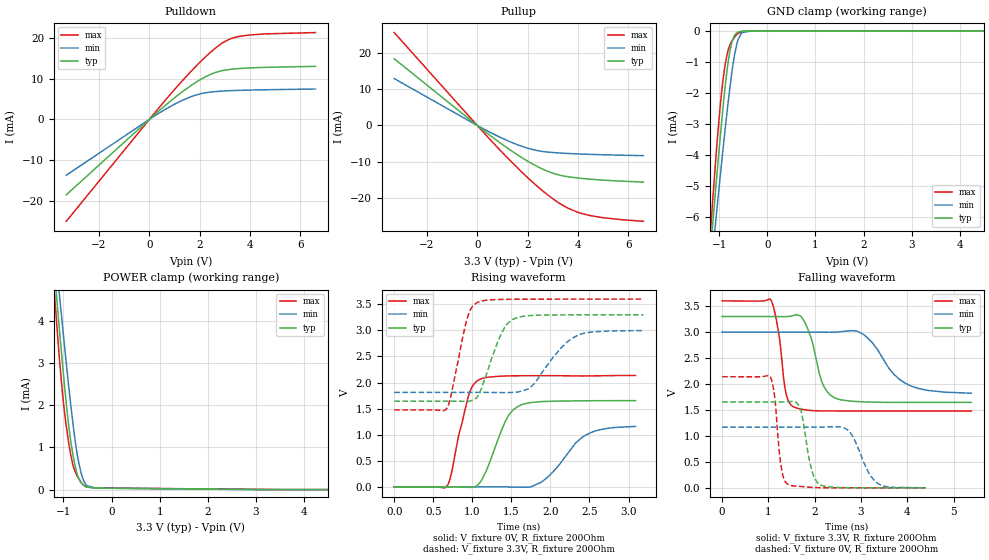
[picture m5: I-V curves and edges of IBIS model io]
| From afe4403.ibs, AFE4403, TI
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|   io Model
[Model]   io
Model_type   I/O
Polarity   Non-Inverting
Enable   Active-Low
Vinl = 0.66
Vinh = 2.64
Vmeas = 1.65
Vref = 0
Cref = 2pF
Rref = 370
|   typ   min   max
|   (nom PVT)   (fast PVT)   (slow PVT)
C_comp   3.788e-13   3.524e-13   3.882e-13
[Model spec]
|subparameter
Vinl   0.66   0.6   0.72
Vinh   2.64   2.4   2.88
| Where nom  PVT is Nominal Process, 3.3V, 27C
|   Fast PVT is Strong Process,  3.6V, -40C
|   Slow PVT is Weak Process,   3V, 105C
[Voltage Range]   3.3   3   3.6
|Junction Temperature
[Temperature Range]   27   105   -40
[Pullup Reference]   3.3   3   3.6
[Pulldown Reference]   0   0   0
[Power Clamp Reference]   3.3   3   3.6
[GND Clamp Reference]   0   0   0
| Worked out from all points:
|   slope of the pulldown table from 0 to 0.495 V, typ, clamps not added: 183 ohm
|   slope of the pullup table from 0 to 0.495 V, typ, clamps not added: 186 ohm
|   GND clamp passes 1 mA (typ) near -0.81 V on its own axis
|   POWER clamp passes 1 mA (typ) near -0.83 V on its own axis
|   falling waveform, V_fixture 3.3V, R_fixture 200Ohm: 20-80 % time 299ps typ, 612ps min, 179ps max; typ from 3.3 V to 1.65 V
|   rising waveform, V_fixture 0V, R_fixture 200Ohm: 20-80 % time 262ps typ, 392ps min, 189ps max; typ from 0 V to 1.65 V
|   rising waveform, V_fixture 3.3V, R_fixture 200Ohm: 20-80 % time 245ps typ, 372ps min, 177ps max; typ from 1.64 V to 3.3 V
|   falling waveform, V_fixture 0V, R_fixture 200Ohm: 20-80 % time 200ps typ, 352ps min, 133ps max; typ from 1.65 V to 0 V
[Pulldown]
|   Voltage   I(typ)   I(min)   I(max)
-3.3V     -18.51mA   -13.7mA    -25.02mA
63mV      352.9uA    259.5uA    478.3uA
821.7mV   4.409mA    3.145mA    6.077mA
1.296V    6.722mA    4.658mA    9.403mA
1.725V    8.612mA    5.747mA    12.26mA
2.237V    10.51mA    6.554mA    15.41mA
2.649V    11.59mA    6.86mA     17.64mA
3.122V    12.22mA    7.045mA    19.54mA
3.633V    12.53mA    7.161mA    20.46mA
4.609V    12.8mA     7.286mA    21.01mA
6.6V      13.04mA    7.482mA    21.34mA
[GND Clamp]
|   Voltage   I(typ)   I(min)   I(max)
-3.3V     -49.34mA   -43.13mA   -58.15mA
-1.216V   -7.733mA   -8.404mA   -7.228mA
-1.158V   -6.649mA   -7.482mA   -5.945mA
-1.143V   -6.369mA   -7.243mA   -5.618mA
-1.066V   -4.952mA   -6.026mA   -3.997mA
-985.2mV  -3.524mA   -4.778mA   -2.503mA
-888mV    -1.953mA   -3.328mA   -1.197mA
-808.8mV  -941.7uA   -2.222mA   -585.8uA
-741mV    -391.7uA   -1.375mA   -342uA
-607.2mV  -38.31uA   -270.4uA   -81.8uA
-330mV    -3.295uA   -3.637uA   -3.333uA
6.6V      0A         0A         0A
[Pullup]
|   Voltage   I(typ)   I(min)   I(max)
-3.3V     18.32mA    12.88mA    25.52mA
0V        0A         0A         0A
877.8mV   -4.633mA   -3.14mA    -6.576mA
1.52V     -7.721mA   -5.078mA   -11.12mA
2.032V    -9.922mA   -6.294mA   -14.52mA
2.442V    -11.46mA   -6.968mA   -17.05mA
2.904V    -12.86mA   -7.37mA    -19.62mA
3.282V    -13.65mA   -7.563mA   -21.44mA
3.627V    -14.1mA    -7.697mA   -22.79mA
4.151V    -14.55mA   -7.856mA   -24.19mA
5.022V    -15.02mA   -8.05mA    -25.35mA
6.6V      -15.54mA   -8.287mA   -26.32mA
[POWER Clamp]
|   Voltage   I(typ)   I(min)   I(max)
-3.3V     35.6mA     31.69mA    41.16mA
-1.183V   5.11mA     5.779mA    4.576mA
-1.098V   3.974mA    4.776mA    3.298mA
-1.079V   3.723mA    4.553mA    3.028mA
-1.018V   2.944mA    3.848mA    2.251mA
-954mV    2.184mA    3.134mA    1.614mA
-870mV    1.327mA    2.231mA    959.3uA
-798mV    791.7uA    1.522mA    558.7uA
-716.1mV  373.3uA    851.9uA    326.4uA
-639mV    169.7uA    418uA      180.9uA
-522mV    62.07uA    96.11uA    61.86uA
6.6V      0A         0A         0A
[Ramp]
R_load = 200
|   typ   min   max
dV/dt_r   0.99127/2.59914e-10   0.701428/3.944e-10   1.28069/1.88964e-10
dV/dt_f   0.991011/2.9628e-10   0.710826/6.13815e-10   1.2707/1.76626e-10
[Falling Waveform]
V_fixture = 3.3V
V_fixture_min = 3V
V_fixture_max = 3.6V
R_fixture = 200Ohm
|   Time   V(typ)   V(min)   V(max)
0s        3.3V       3V         3.6V
1.054ns   3.297V     2.996V     3.613V
1.384ns   3.296V     2.996V     1.8V
1.514ns   3.312V     2.996V     1.571V
1.792ns   3.174V     2.997V     1.502V
2.168ns   2.013V     2.995V     1.48V
2.43ns    1.732V     2.997V     1.48V
3.046ns   1.655V     2.956V     1.48V
4.062ns   1.645V     1.966V     1.479V
5.38ns    1.645V     1.823V     1.479V
[Rising Waveform]
V_fixture = 0V
V_fixture_min = 0V
V_fixture_max = 0V
R_fixture = 200Ohm
|   Time   V(typ)   V(min)   V(max)
0s        3.314nV    8.702nV    2.857nV
682ps     50.52uV    2.115uV    29.33mV
732ps     427uV      2.27uV     258.5mV
948ps     -6.572mV   -23.93uV   1.729V
1.104ns   97.84mV    14.7uV     2.067V
1.42ns    1.251V     288.3uV    2.125V
1.578ns   1.538V     -4.621mV   2.129V
1.932ns   1.637V     145.2mV    2.132V
2.502ns   1.651V     1.032V     2.126V
3.09ns    1.652V     1.159V     2.135V
[Rising Waveform]
V_fixture = 3.3V
V_fixture_min = 3V
V_fixture_max = 3.6V
R_fixture = 200Ohm
|   Time   V(typ)   V(min)   V(max)
0s        1.643V     1.811V     1.475V
672ps     1.643V     1.811V     1.502V
934ps     1.642V     1.811V     3.223V
1.07ns    1.738V     1.812V     3.535V
1.332ns   2.803V     1.808V     3.59V
1.514ns   3.206V     1.811V     3.595V
1.73ns    3.281V     1.887V     3.596V
2.132ns   3.295V     2.655V     3.597V
2.362ns   3.296V     2.914V     3.597V
3.19ns    3.297V     2.995V     3.597V
[Falling Waveform]
V_fixture = 0V
V_fixture_min = 0V
V_fixture_max = 0V
R_fixture = 200Ohm
|   Time   V(typ)   V(min)   V(max)
0s        1.654V     1.169V     2.139V
1.036ns   1.654V     1.169V     2.143V
1.264ns   1.654V     1.169V     472.3mV
1.398ns   1.657V     1.169V     81.98mV
1.692ns   1.523V     1.169V     27.24mV
1.908ns   434.4mV    1.169V     10.48mV
2.128ns   53.03mV    1.169V     2.925mV
2.762ns   2.002mV    1.069V     248.9uV
3.364ns   170.1uV    82.74mV    82.22uV
4.39ns    69.86uV    1.951mV    37.89uV
